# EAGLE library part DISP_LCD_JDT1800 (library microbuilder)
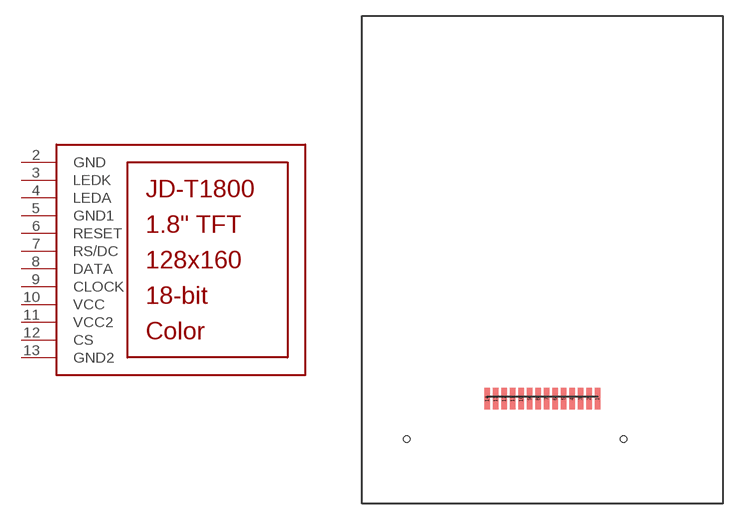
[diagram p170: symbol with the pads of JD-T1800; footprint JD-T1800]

Designator prefix LCD

## DISP_LCD_JDT1800  [JD-T1800]
2  GND  pwr
3  LEDK  in
4  LEDA  in
5  GND1  pwr
6  RESET  in
7  RS/DC  in
8  DATA
9  CLOCK  in
10  VCC  pwr
11  VCC2  pwr
12  CS  in
13  GND2  pwr

## Footprint JD-T1800 (pad centres in mm)
smd 0.5 x 2: 1 5.2,-13.1; 2 4.4,-13.1; 3 3.6,-13.1; 4 2.8,-13.1; 5 2,-13.1; 6 1.2,-13.1; 7 0.4,-13.1; 8 -0.4,-13.1; 9 -1.2,-13.1; 10 -2,-13.1; 11 -2.8,-13.1; 12 -3.6,-13.1; 13 -4.4,-13.1; 14 -5.2,-13.1
hole 0.6 at -12.8,-16.9
hole 0.6 at 7.65,-16.9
